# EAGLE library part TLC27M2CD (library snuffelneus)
DUAL OPERATIONAL AMPLIFIERS
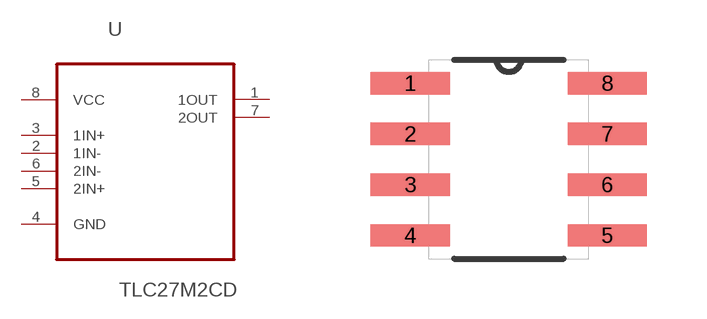
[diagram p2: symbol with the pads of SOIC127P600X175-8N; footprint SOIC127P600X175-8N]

Designator prefix U

## TLC27M2CD (MPN: TLC27M2CD; OC_FARNELL: 1470381; OC_NEWARK: 67K1260; PACKAGE: SOIC-8; SUPPLIER: Texas Instruments)  [SOIC127P600X175-8N]
1  1OUT  out
2  1IN-  in
3  1IN+  in
4  GND  pas
5  2IN+  in
6  2IN-  in
7  2OUT  out
8  VCC  pwr

## Footprint SOIC127P600X175-8N (pad centres in mm)
smd 1.981 x 0.559: 1 -2.464,1.905; 2 -2.464,0.635; 3 -2.464,-0.635; 4 -2.464,-1.905; 5 2.464,-1.905; 6 2.464,-0.635; 7 2.464,0.635; 8 2.464,1.905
